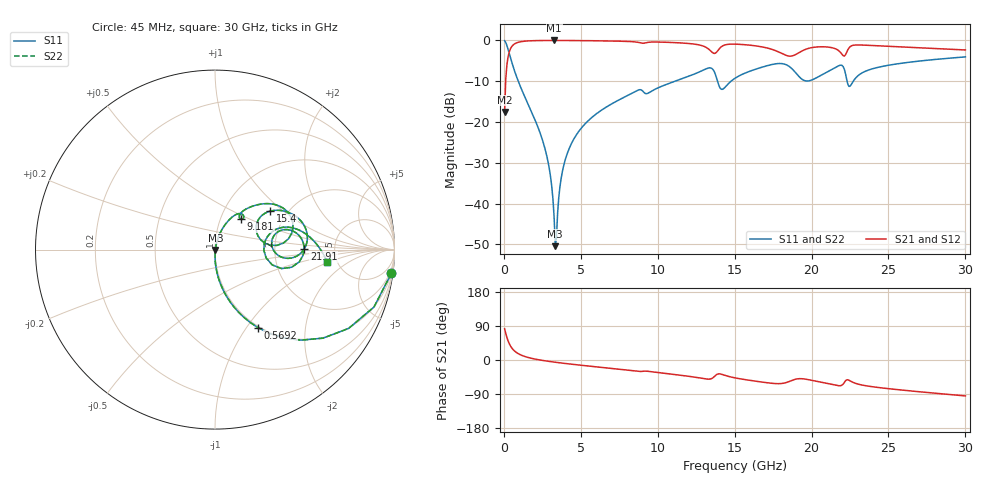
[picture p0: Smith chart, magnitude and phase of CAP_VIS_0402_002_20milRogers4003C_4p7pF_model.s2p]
! S-parameter model data by Modelithics Inc.  support@modelithics.com  813-866-6335  Tampa FL USA
! S-Parameter data specifications:
! Substrate: 20-mil Rogers 4003C, substrate thickness, H=0.508mm, Dielectric constant, Er=3.75
! PCB Mounting Pad Footprint: Pad width, PadW=0.50mm , Pad length, PadL=0.50mm , Pad gap, PadG (edge-to-edge)=0.40mm , Reference planes=1.4mm apart
! Created Wed Nov 18 12:47:51 2015
# hz S ma R 50
! 2 Port Network Data from SP1.SP block
! freq  magS11  angS11  magS21  angS21  magS12  angS12  magS22  angS22
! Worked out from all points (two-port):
!   401 points, 45 MHz to 30 GHz, reference 50 ohm
!   highest |S21| = -0.02 dB at 3.265 GHz (marker M1); lowest = -17.5 dB at 45 MHz (marker M2)
!   |S21| within 3 dB of the highest: 334.6 MHz to 13.57 GHz (13.24 GHz wide, 190 % of centre); 22.27 GHz to end of sweep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
!   lowest |S11| = -50.4 dB at 3.34 GHz (marker M3), VSWR 1.01, Z = 50.2 - j0.193 ohm
!   |S11| at or under -10 dB: 931.4 MHz to 11.14 GHz (10.21 GHz wide, 169 % of centre); 13.89 GHz to 14.77 GHz (883.4 MHz wide, 6.17 % of centre); 22.31 GHz to 22.71 GHz (404.3 MHz wide, 1.8 % of centre)
!   |S22| runs from -50.4 to -0.1 dB; largest |S21 - S12| = 0
!   S11 on the Smith chart (normalised r, x): 45 MHz: 1, -15; 569.2 MHz: 0.98, -1.14; 9.181 GHz: 1.26, +0.45; 15.4 GHz: 1.64, +0.82; 21.91 GHz: 2.98, +0.03; 30 GHz: 4.15, -0.92
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4.5e7  0.9912 -7.7  0.1327 82.3  0.1327 82.3  0.9912 -7.7
2.696625e8  0.778 -39.4  0.6278 50.6  0.6278 50.6  0.778 -39.4
5.692125e8  0.4975 -61.1  0.8665 28.8  0.8665 28.8  0.4975 -61.1
1.168312e9  0.2454 -77.6  0.9679 12.1  0.9679 12.1  0.2454 -77.6
2.666062e9  0.04731 -89.4  0.9966 -2.1  0.9966 -2.1  0.04731 -89.4
3.0405e9  0.02073 -87.7  0.9973 -4.3  0.9973 -4.3  0.02073 -87.7
3.265162e9  0.006707 -74.0  0.9974 -5.6  0.9974 -5.6  0.006707 -74.0
3.34005e9  0.003003 -39.8  0.9974 -6.0  0.9974 -6.0  0.003003 -39.8
4.014038e9  0.03579 76.3  0.9965 -9.3  0.9965 -9.3  0.03579 76.3
5.062462e9  0.0854 73.8  0.993 -14.1  0.993 -14.1  0.0854 73.8
9.181275e9  0.2238 49.1  0.9302 -29.3  0.9302 -29.3  0.2238 49.1
1.007992e10  0.265 54.1  0.9532 -33.6  0.9532 -33.6  0.265 54.1
1.344986e10  0.459 19.5  0.7403 -49.8  0.7403 -49.8  0.459 19.5
1.412385e10  0.2518 17.0  0.832 -37.4  0.832 -37.4  0.2518 17.0
1.50225e10  0.3432 36.0  0.899 -47.2  0.899 -47.2  0.3432 36.0
1.539694e10  0.376 34.8  0.8921 -49.9  0.8921 -49.9  0.376 34.8
1.8018e10  0.52 8.4  0.6977 -62.1  0.6977 -62.1  0.52 8.4
2.003996e10  0.3284 11.5  0.8168 -53.9  0.8168 -53.9  0.3284 11.5
2.191215e10  0.497 0.4  0.7 -67.5  0.7 -67.5  0.497 0.4
2.251125e10  0.2758 6.3  0.8378 -55.2  0.8378 -55.2  0.2758 6.3
2.505742e10  0.4976 11.5  0.844 -75.9  0.844 -75.9  0.4976 11.5
3e10  0.627 -6.2  0.7627 -94.8  0.7627 -94.8  0.627 -6.2
